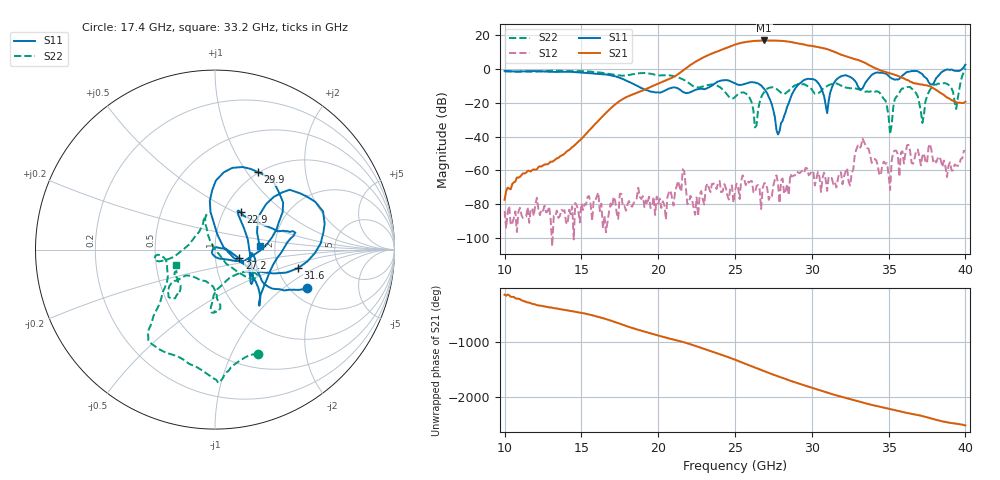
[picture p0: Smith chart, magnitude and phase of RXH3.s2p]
!Keysight Technologies,M9808A,MY58100618,A.14.70.03
!Date: Monday, February 27, 2023 13:43:21
!Correction: S11(Cdelta 2-Port  )
!S21(Cdelta 2-Port  )
!S12(Cdelta 2-Port  )
!S22(Cdelta 2-Port  )
!S2P File: Measurements: S11, S21, S12, S22:
# Hz S  RI  R 50
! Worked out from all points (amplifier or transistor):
!   301 points, 10 GHz to 40 GHz, reference 50 ohm
!   highest |S21| = 16.6 dB at 26.9 GHz (marker M1)
!   |S21| within 3 dB of that: 24.82 GHz to 29.78 GHz (4.957 GHz wide, 18.2 % of centre)
!   unconditionally stable (mu >= 1): start of sweep to 39.82 GHz
!   at 15 GHz: K = 65600.16, MAG = -32.2 dB, |S12| = -79.3 dB
!   at 25 GHz: K = 330.82, MAG = 14.9 dB, |S12| = -72.0 dB
!   at 40 GHz: K = 14.86, MSG = 14.5 dB, |S12| = -48.4 dB
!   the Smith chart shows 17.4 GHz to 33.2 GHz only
!   S11 on the Smith chart (normalised r, x): 17.4 GHz: 2.42, -1.50; 22.9 GHz: 1.21, +0.54; 27.2 GHz: 1.31, -0.13; 29.9 GHz: 0.99, +1.13; 31.6 GHz: 2.58, -0.69; 33.2 GHz: 1.66, +0.07
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1e10  0.0316 0.8584  -0.000127 -5.31e-05  6.39e-05 -8.36e-06  0.7477 0.3343
1.5e10  0.7282 0.2224  -0.00475 -0.00707  -9.29e-05 5.55e-05  0.6112 -0.5821
1.74e10  0.5102 -0.2153  0.0648 0.0807  3.47e-05 -1.45e-05  0.2408 -0.5827
2e10  0.1971 -0.0369  -0.3565 -0.0537  6.16e-06 -0.000106  -0.1754 -0.613
2.29e10  0.144 0.2081  1.506 -1.44  0.000103 9.4e-05  -0.297 -0.0368
2.39e10  0.4035 0.1025  -2.439 -2.157  0.000262 -0.000349  -0.2966 -0.0628
2.45e10  0.4447 0.0905  -4.006 1.089  -3.95e-05 0.00018  -0.171 0.00565
2.5e10  0.3694 -0.0161  -2.001 4.686  -0.00018 -0.000175  -0.0754 0.1246
2.55e10  0.2748 -0.1983  3.076 4.973  -0.000312 -0.00065  -0.0484 0.1942
2.6e10  0.246 -0.3119  6.284 0.3781  -0.000461 -0.000139  -0.0459 0.1166
2.69e10  0.2056 -0.1459  -0.5018 -6.719  -0.000368 0.000202  0.1487 -0.1372
2.72e10  0.1362 -0.0489  -3.937 -5.457  -5.12e-05 -0.000127  0.2179 -0.1599
2.78e10  -0.00625 0.00962  -6.534 0.8378  -0.000142 -0.000394  0.1974 -0.1249
2.85e10  0.078 -0.0567  -1.438 6.045  7.09e-05 0.000174  0.0121 -0.221
2.93e10  0.3558 0.1528  4.652 2.64  -0.000907 0.000127  -0.00237 -0.3429
2.99e10  0.2387 0.4323  4.335 -1.853  -0.000243 0.000765  0.0118 -0.2747
3e10  0.1969 0.4503  3.988 -2.432  -0.000381 0.000878  0.00749 -0.2419
3.07e10  -0.0251 0.2094  -0.2278 -4.057  0.000207 0.000568  -0.1923 -0.1601
3.16e10  0.4611 -0.1046  -2.91 -0.5017  -8.09e-05 0.000306  -0.2463 -0.2722
3.32e10  0.2486 0.0191  0.5756 1.555  -0.000672 -0.00504  -0.2164 -0.0881
3.5e10  0.5877 0.1637  0.4758 -0.5679  0.0007 0.000197  -0.0382 -6.73e-05
4e10  1.192 -0.5356  0.1046 0.0147  0.00284 -0.00249  0.4634 -0.8961
